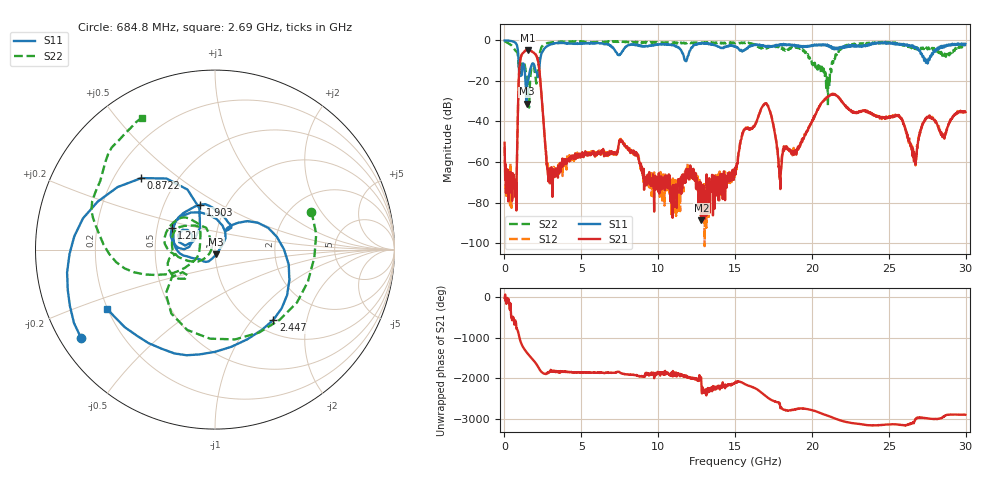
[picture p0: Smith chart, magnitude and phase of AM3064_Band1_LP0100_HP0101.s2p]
# Hz S DB R 50.0
!freq dBS11 angS11 dBS21 angS21 dBS12 angS12 dBS22 angS22
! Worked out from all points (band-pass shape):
!   1600 points, 10 MHz to 29.98 GHz, reference 50 ohm
!   highest |S21| = -4.69 dB at 1.528 GHz (marker M1); lowest = -88.8 dB at 12.81 GHz (marker M2)
!   |S21| within 3 dB of the highest: 1.09 GHz to 2.083 GHz (992.2 MHz wide, 62.5 % of centre)
!   lowest |S11| = -31.3 dB at 1.435 GHz (marker M3), VSWR 1.06, Z = 50.6 - j2.68 ohm
!   |S11| at or under -10 dB: 916.7 MHz to 2.314 GHz (1.397 GHz wide, 86.5 % of centre); 11.75 GHz to 11.84 GHz (89.15 MHz wide, 0.756 % of centre); 27.4888 GHz to 27.56452 GHz (75.72 MHz wide, 0.275 % of centre)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
!   |S22| runs from -33.2 to -0.4 dB; largest |S21 - S12| = 0.0073
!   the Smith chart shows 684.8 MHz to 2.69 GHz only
!   S11 on the Smith chart (normalised r, x): 684.8 MHz: 0.06, -0.30; 872.2 MHz: 0.31, +0.37; 1.21 GHz: 0.60, +0.16; 1.903 GHz: 0.75, +0.41; 2.447 GHz: 1.22, -1.29; 2.69 GHz: 0.20, -0.25
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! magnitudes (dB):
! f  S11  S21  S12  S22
! 10 MHz  -0.1  -50.5  -52.7  -0.4
! 684.8 MHz  -1.0  -73.3  -69.8  -4.8
! 872.2 MHz  -4.8  -36.3  -36.2  -7.3
! 1.21 GHz  -11.4  -6.2  -6.1  -10.8
! 1.435 GHz  -31.3  -4.8  -4.8  -17.3
! 1.528 GHz  -20.3  -4.7  -4.6  -22.3
! 1.903 GHz  -11.6  -6.1  -6.0  -12.6
! 2.447 GHz  -5.9  -30.9  -30.8  -2.8
! 2.69 GHz  -3.3  -55.1  -56.1  -1.5
! 5.015 GHz  -1.5  -57.1  -56.0  -0.6
! 7.62 GHz  -6.0  -49.5  -49.4  -0.7
! 10 GHz  -2.0  -67.5  -71.7  -0.9
! 12.81 GHz  -1.5  -88.8  -74.2  -1.2
! 15 GHz  -3.2  -64.2  -66.0  -1.4
! 16.92 GHz  -2.8  -31.3  -31.3  -3.9
! 17.93 GHz  -2.0  -68.0  -65.2  -3.1
! 19.99 GHz  -2.8  -40.0  -40.2  -11.1
! 21.34 GHz  -3.9  -26.4  -26.6  -10.6
! 25 GHz  -1.1  -38.0  -37.4  -1.1
! 26.68 GHz  -3.1  -56.4  -58.9  -4.2
! 27.49 GHz  -10.0  -37.7  -38.2  -4.0
! 29.98 GHz  -1.7  -35.4  -35.5  -2.8
